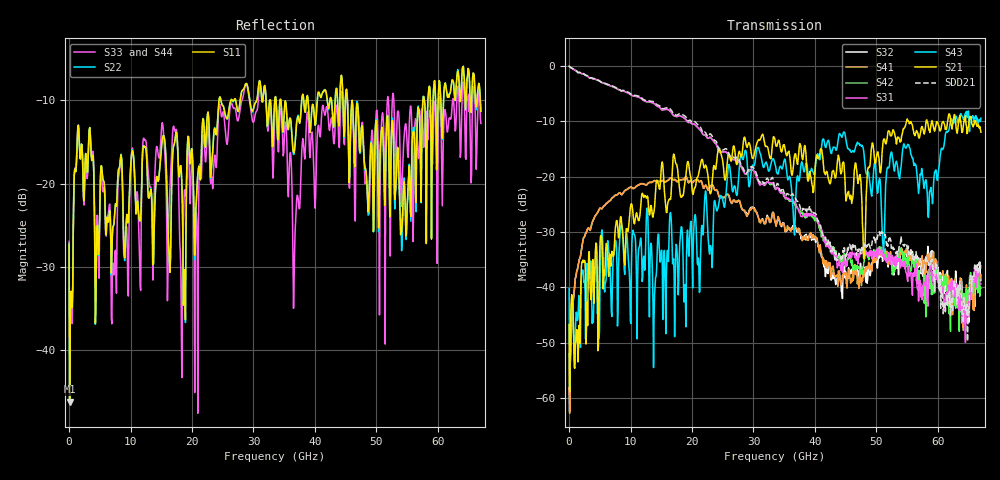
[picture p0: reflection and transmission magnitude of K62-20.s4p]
!Agilent Technologies,N5247A,US50470101,A.10.25.02
!Agilent N5247A: A.10.25.02
!Date: Tuesday, May 12, 2015 13:41:03
!Correction: Sdd11(Full 4 Port(1,2,3,4))
!Sdc11(Full 4 Port(1,2,3,4))
!Sdd12(Full 4 Port(1,2,3,4))
!Sdc12(Full 4 Port(1,2,3,4))
!Scd11(Full 4 Port(1,2,3,4))
!Scc11(Full 4 Port(1,2,3,4))
!Scd12(Full 4 Port(1,2,3,4))
!Scc12(Full 4 Port(1,2,3,4))
!Sdd21(Full 4 Port(1,2,3,4))
!Sdc21(Full 4 Port(1,2,3,4))
!Sdd22(Full 4 Port(1,2,3,4))
!Sdc22(Full 4 Port(1,2,3,4))
!Scd21(Full 4 Port(1,2,3,4))
!Scc21(Full 4 Port(1,2,3,4))
!Scd22(Full 4 Port(1,2,3,4))
!Scc22(Full 4 Port(1,2,3,4))
!Balanced Topology: BBAL
!S4P File: Measurements: <Sdd11,Sdc11,Sdd12,Sdc12>,
!<Scd11,Scc11,Scd12,Scc12>,
!<Sdd21,Sdc21,Sdd22,Sdc22>,
!<Scd21,Scc21,Scd22,Scc22>:
# Hz S  dB  R 50
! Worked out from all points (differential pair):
!   801 points, 10 MHz to 67 GHz, reference 50 ohm
!   strongest paths, dB at 10 MHz, 16.76 GHz, 33.51 GHz, 50.25 GHz, 67 GHz:
!     S21: -46.7, -19.5, -13.4, -15.5, -12.0
!     S43: -40.2, -32.0, -17.7, -22.8, -9.4
!     S31: 0.0, -8.6, -22.0, -32.9, -39.4
!     S42: 0.0, -8.6, -22.2, -33.0, -40.2
!     S41: -52.0, -20.4, -28.2, -34.4, -37.7
!     S32: -58.1, -20.4, -28.2, -35.6, -38.7
!   taken as a pair (ports 1,2 in; 3,4 out), SDD21 dB: 0.0, -8.2, -22.0, -30.5, -36.0
!   lowest |S11| = -46.2 dB at 93.74 MHz (marker M1), VSWR 1.01, Z = 49.7 - j0.409 ohm
!   |S11| at or under -10 dB: start of sweep to 24.41 GHz; 34.45 GHz to 37.86 GHz (3.411 GHz wide, 9.44 % of centre); 46.07 GHz to 57.58 GHz (11.51 GHz wide, 22.2 % of centre)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
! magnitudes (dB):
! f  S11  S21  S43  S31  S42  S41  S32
! 10 MHz  -27.3  -46.7  -40.2  0.0  0.0  -52.0  -58.1
! 93.74 MHz  -46.2  -58.9  -57.8  -0.1  -0.1  -62.8  -62.4
! 2.606 GHz  -17.6  -35.5  -40.9  -1.6  -1.6  -30.5  -30.4
! 11.65 GHz  -24.3  -25.4  -31.1  -5.8  -5.8  -21.3  -21.3
! 31.33 GHz  -9.8  -12.6  -16.9  -21.2  -21.3  -27.8  -27.9
! 47.99 GHz  -17.0  -34.9  -15.9  -34.1  -35.3  -38.0  -37.1
! 67 GHz  -11.3  -12.0  -9.4  -39.4  -40.2  -37.7  -38.7
